FUNCTION "ASSE Z" : VOID
TITLE =GESTIONE SEGNALI DI STATO E COMANDO DELL'ASSE Z
VERSION : 0.1

BEGIN
NETWORK
TITLE =INS./DISIN.1
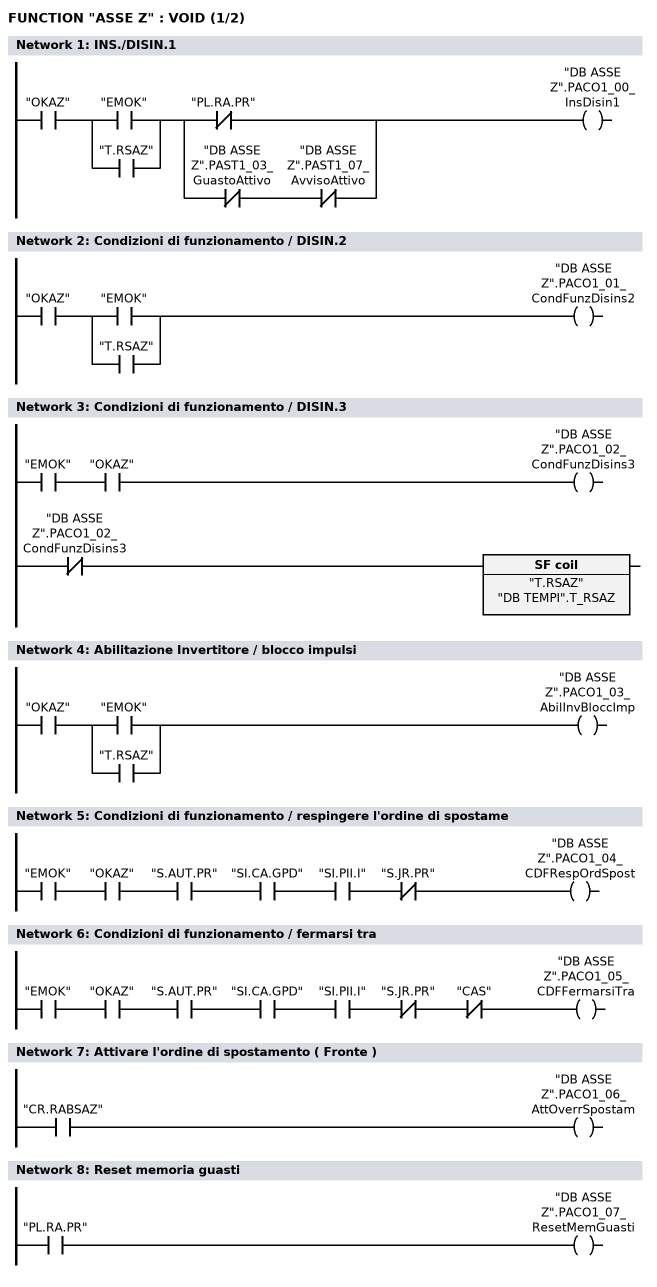
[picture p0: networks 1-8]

      U     "OKAZ";
      U(    ;
      O     "EMOK";
      O     "T.RSAZ";
      )     ;
      U(    ;
      UN    "PL.RA.PR";
      O     ;
      UN    "DB ASSE Z".PAST1_03_GuastoAttivo;
      UN    "DB ASSE Z".PAST1_07_AvvisoAttivo;
      )     ;
      =     "DB ASSE Z".PACO1_00_InsDisin1;

NETWORK
TITLE =Condizioni di funzionamento / DISIN.2

      U     "OKAZ";
      U(    ;
      O     "EMOK";
      O     "T.RSAZ";
      )     ;
      =     "DB ASSE Z".PACO1_01_CondFunzDisins2;

NETWORK
TITLE =Condizioni di funzionamento / DISIN.3

      U     "EMOK";
      U     "OKAZ";
      =     "DB ASSE Z".PACO1_02_CondFunzDisins3;
//---------------------------
      UN    "DB ASSE Z".PACO1_02_CondFunzDisins3;
      L     "DB TEMPI".T_RSAZ;
      SA    "T.RSAZ";

NETWORK
TITLE =Abilitazione Invertitore / blocco impulsi

      U     "OKAZ";
      U(    ;
      O     "EMOK";
      O     "T.RSAZ";
      )     ;
      =     "DB ASSE Z".PACO1_03_AbilInvBloccImp;

NETWORK
TITLE =Condizioni di funzionamento / respingere l'ordine di spostame

      U     "EMOK";
      U     "OKAZ";
      U     "S.AUT.PR";
      U     "SI.CA.GPD";
      U     "SI.PII.I";

      UN    "S.JR.PR";
      =     "DB ASSE Z".PACO1_04_CDFRespOrdSpost;

NETWORK
TITLE =Condizioni di funzionamento / fermarsi tra

      U     "EMOK";
      U     "OKAZ";
      U     "S.AUT.PR";
      U     "SI.CA.GPD";
      U     "SI.PII.I";
      UN    "S.JR.PR";

      UN    "CAS";
      =     "DB ASSE Z".PACO1_05_CDFFermarsiTra;

NETWORK
TITLE =Attivare l'ordine di spostamento ( Fronte )

      U     "CR.RABSAZ";
      =     "DB ASSE Z".PACO1_06_AttOverrSpostam;

NETWORK
TITLE =Reset memoria guasti

      U     "PL.RA.PR";
      =     "DB ASSE Z".PACO1_07_ResetMemGuasti;

NETWORK
TITLE =Marcia impulsi 1 INS
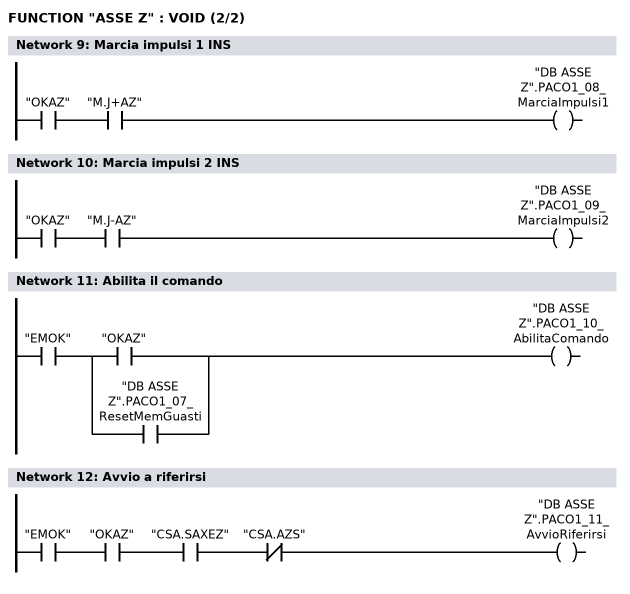
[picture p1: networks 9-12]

      U     "OKAZ";
      U     "M.J+AZ";
      =     "DB ASSE Z".PACO1_08_MarciaImpulsi1;

NETWORK
TITLE =Marcia impulsi 2 INS

      U     "OKAZ";
      U     "M.J-AZ";
      =     "DB ASSE Z".PACO1_09_MarciaImpulsi2;

NETWORK
TITLE =Abilita il comando

      U     "EMOK";
      U(    ;
      U     "OKAZ";
      O     ;
      U     "DB ASSE Z".PACO1_07_ResetMemGuasti;
      )     ;
      =     "DB ASSE Z".PACO1_10_AbilitaComando;

NETWORK
TITLE =Avvio a riferirsi

      U     "EMOK";
      U     "OKAZ";
      U     "CSA.SAXEZ";
      UN    "CSA.AZS";
      =     "DB ASSE Z".PACO1_11_AvvioRiferirsi;

NETWORK
TITLE =Cambio del blocco esterno

      CLR   ;
      =     "DB ASSE Z".PACO1_13_CambioBloccoExt;

NETWORK
TITLE =Caricamento del numero blocco di spostamento desiderato



NETWORK
TITLE =Funzionamento a seguire
//
      CLR   ;
      =     "DB ASSE Z".POSPACO_00_FunzASeguire;

NETWORK
TITLE =Imposta il punto di riferimento

      CLR   ;
      =     "DB ASSE Z".POSPACO_01_ImpostPuntRif;

NETWORK
TITLE =Camma di riferimento

      UN    "FC.ZAZ";
      =     "DB ASSE Z".POSPACO_02_CammaRiferime;

NETWORK
TITLE =Sensore della battuta fissa

      CLR   ;
      =     "DB ASSE Z".POSPACO_03_SensBattFissa;

NETWORK
TITLE =Attivare l'accoppiamento

      CLR   ;
      =     "DB ASSE Z".POSPACO_04_AttivAccoppia;

NETWORK
TITLE =Commutazione del blocco di parametri Bit 0

      CLR   ;
      =     "DB ASSE Z".PACO2_00_CommBlocParBit1;


NETWORK
TITLE =Commutazione del blocco di parametri Bit 1

      CLR   ;
      =     "DB ASSE Z".PACO2_01_CommBlocParBit2;

NETWORK
TITLE =Commutazione del blocco di parametri Bit 2

      CLR   ;
      =     "DB ASSE Z".PACO2_02_CommBlocParBit3;

NETWORK
TITLE =Primo filtro nel riferimento di velocita' disinserito
//
      CLR   ;
      =     "DB ASSE Z".PACO2_03_1FiltRifVelDisi;

NETWORK
TITLE =Tempo rampa zero

      CLR   ;
      =     "DB ASSE Z".PACO2_04_TempoRampaZero;

NETWORK
TITLE =Blocco dell'integratore nel regolatore di velocita'

      CLR   ;
      =     "DB ASSE Z".PACO2_06_BlocIntegrRegV;

NETWORK
TITLE =Scelta dell'asse in parcheggio

      CLR   ;
      =     "DB ASSE Z".PACO2_07_SceltaAsseInPar;

NETWORK
TITLE =Tacitare il guasto 608

      U     "OKAZ";
      U     "PL.RA.PR";
      =     "DB ASSE Z".PACO2_08_TacitGuasto608;

NETWORK
TITLE =Commutazione dati del motore 1 ingresso

      CLR   ;
      =     "DB ASSE Z".PACO2_09_CommDatiMot1Ing;

NETWORK
TITLE =Commutazione dati del motore 2 ingresso

      CLR   ;
      =     "DB ASSE Z".PACO2_10_CommDatiMot2Ing;

NETWORK
TITLE =Ha luogo la ommutazione del motore

      CLR   ;
      =     "DB ASSE Z".PACO2_11_CommutazMotore;

NETWORK
TITLE =OVERRIDE

      U     "M.MAN";
      UN    "P.JR.PR";
      SPBN  E001;
      L     "DB DATI".OVERRIDE_JOG;
      T     "DB ASSE Z".OVERRIDE;
      T     "DB DATI".OVERRIDE_ATTIVO;
E001: NOP   0;
      U     "M.MAN";
      U     "P.JR.PR";
      SPBN  E002;
      L     "DB DATI".OVERRIDE_JOG;
      L     2;
      *I    ;
      T     "DB ASSE Z".OVERRIDE;
      T     "DB DATI".OVERRIDE_ATTIVO;
E002: NOP   0;
      UN    "M.MAN";
      SPBN  E003;
      L     "DB DATI".OVERRIDE_AUT;
      T     "DB ASSE Z".OVERRIDE;
      T     "DB DATI".OVERRIDE_ATTIVO;
E003: NOP   0;

NETWORK
TITLE =Caricamento quote

      U     "ANSD";
      UN    "CQAZ.IC";
      S     "CQAZ.IC";
      S     "CQAZ.Q1";
//============================ QUOTA 1
      U     "CQAZ.Q1";
      SPBN  ET01;
      L     W#16#8051;
      T     "DB ASSE Z".PKE_Scrittura;
      L     W#16#1;
      T     "DB ASSE Z".IND_Scrittura;
      L     "DB QUOTE".Z_ATTESA;
      T     DB123.DBD    4;
//----------------------------
      U(    ;
      L     "DB ASSE Z".PKE_Lettura;
      L     W#16#5051;
      ==I   ;
      )     ;
      U(    ;
      L     "DB ASSE Z".IND_Lettura;
      L     W#16#1;
      ==I   ;
      )     ;
      R     "CQAZ.Q1";
      S     "CQAZ.Q2";
ET01: NOP   0;
//============================ QUOTA 2
      U     "CQAZ.Q2";
      SPBN  ET02;
      L     W#16#8051;
      T     "DB ASSE Z".PKE_Scrittura;
      L     W#16#2;
      T     "DB ASSE Z".IND_Scrittura;
      L     "DB QUOTE".Z_FUORI_INGOMBRO;
      T     DB123.DBD    4;
//----------------------------
      U(    ;
      L     "DB ASSE Z".PKE_Lettura;
      L     W#16#5051;
      ==I   ;
      )     ;
      U(    ;
      L     "DB ASSE Z".IND_Lettura;
      L     W#16#2;
      ==I   ;
      )     ;
      R     "CQAZ.Q2";
      S     "CQAZ.Q3";
ET02: NOP   0;
//============================ QUOTA 3
      U     "CQAZ.Q3";
      SPBN  ET03;
      L     W#16#8051;
      T     "DB ASSE Z".PKE_Scrittura;
      L     W#16#3;
      T     "DB ASSE Z".IND_Scrittura;
      L     "DB QUOTE".Z_DEPOSITO1;
      T     DB123.DBD    4;
//----------------------------
      U(    ;
      L     "DB ASSE Z".PKE_Lettura;
      L     W#16#5051;
      ==I   ;
      )     ;
      U(    ;
      L     "DB ASSE Z".IND_Lettura;
      L     W#16#3;
      ==I   ;
      )     ;
      R     "CQAZ.Q3";
      S     "CQAZ.Q4";
ET03: NOP   0;
//============================ QUOTA 4
      U     "CQAZ.Q4";
      SPBN  ET04;
      L     W#16#8051;
      T     "DB ASSE Z".PKE_Scrittura;
      L     W#16#4;
      T     "DB ASSE Z".IND_Scrittura;
      L     "DB QUOTE".Z_DEPOSITO2;
      T     DB123.DBD    4;
//----------------------------
      U(    ;
      L     "DB ASSE Z".PKE_Lettura;
      L     W#16#5051;
      ==I   ;
      )     ;
      U(    ;
      L     "DB ASSE Z".IND_Lettura;
      L     W#16#4;
      ==I   ;
      )     ;
      R     "CQAZ.Q4";
      S     "CQAZ.Q5";
ET04: NOP   0;
//============================ QUOTA 5
      U     "CQAZ.Q5";
      SPBN  ET05;
      L     W#16#8051;
      T     "DB ASSE Z".PKE_Scrittura;
      L     W#16#5;
      T     "DB ASSE Z".IND_Scrittura;
      L     "DB QUOTE".Z_DEPOSITO3;
      T     DB123.DBD    4;
//----------------------------
      U(    ;
      L     "DB ASSE Z".PKE_Lettura;
      L     W#16#5051;
      ==I   ;
      )     ;
      U(    ;
      L     "DB ASSE Z".IND_Lettura;
      L     W#16#5;
      ==I   ;
      )     ;
      R     "CQAZ.Q5";
      S     "CQAZ.Q6";
ET05: NOP   0;
//============================ QUOTA 6
      U     "CQAZ.Q6";
      SPBN  ET06;
      L     W#16#8051;
      T     "DB ASSE Z".PKE_Scrittura;
      L     W#16#6;
      T     "DB ASSE Z".IND_Scrittura;
      L     "DB QUOTE".Z_DEPOSITO4;
      T     DB123.DBD    4;
//----------------------------
      U(    ;
      L     "DB ASSE Z".PKE_Lettura;
      L     W#16#5051;
      ==I   ;
      )     ;
      U(    ;
      L     "DB ASSE Z".IND_Lettura;
      L     W#16#6;
      ==I   ;
      )     ;
      R     "CQAZ.Q6";
      S     "CQAZ.Q7";
ET06: NOP   0;
//============================ QUOTA 7
      U     "CQAZ.Q7";
      SPBN  ET07;
      L     W#16#8051;
      T     "DB ASSE Z".PKE_Scrittura;
      L     W#16#7;
      T     "DB ASSE Z".IND_Scrittura;
      L     "DB QUOTE".Z_DEPOSITO5;
      T     DB123.DBD    4;
//----------------------------
      U(    ;
      L     "DB ASSE Z".PKE_Lettura;
      L     W#16#5051;
      ==I   ;
      )     ;
      U(    ;
      L     "DB ASSE Z".IND_Lettura;
      L     W#16#7;
      ==I   ;
      )     ;
      R     "CQAZ.Q7";
      S     "CQAZ.Q8";
ET07: NOP   0;
//============================ QUOTA 8
      U     "CQAZ.Q8";
      SPBN  ET08;
      L     W#16#8051;
      T     "DB ASSE Z".PKE_Scrittura;
      L     W#16#8;
      T     "DB ASSE Z".IND_Scrittura;
      L     "DB QUOTE".Z_DEPOSITO6;
      T     DB123.DBD    4;
//----------------------------
      U(    ;
      L     "DB ASSE Z".PKE_Lettura;
      L     W#16#5051;
      ==I   ;
      )     ;
      U(    ;
      L     "DB ASSE Z".IND_Lettura;
      L     W#16#8;
      ==I   ;
      )     ;
      R     "CQAZ.Q8";
      S     "CQAZ.Q9";
ET08: NOP   0;
//============================ QUOTA 9
      U     "CQAZ.Q9";
      SPBN  ET09;
      L     W#16#8051;
      T     "DB ASSE Z".PKE_Scrittura;
      L     W#16#9;
      T     "DB ASSE Z".IND_Scrittura;
      L     "DB QUOTE".Z_DEPOSITO7;
      T     DB123.DBD    4;
//----------------------------
      U(    ;
      L     "DB ASSE Z".PKE_Lettura;
      L     W#16#5051;
      ==I   ;
      )     ;
      U(    ;
      L     "DB ASSE Z".IND_Lettura;
      L     W#16#9;
      ==I   ;
      )     ;
      R     "CQAZ.Q9";
      S     "CQAZ.Q10";
ET09: NOP   0;
//============================ QUOTA 10
      U     "CQAZ.Q10";
      SPBN  ET10;
      L     W#16#8051;
      T     "DB ASSE Z".PKE_Scrittura;
      L     W#16#A;
      T     "DB ASSE Z".IND_Scrittura;
      L     "DB QUOTE".Z_DEPOSITO8;
      T     DB123.DBD    4;
//----------------------------
      U(    ;
      L     "DB ASSE Z".PKE_Lettura;
      L     W#16#5051;
      ==I   ;
      )     ;
      U(    ;
      L     "DB ASSE Z".IND_Lettura;
      L     W#16#A;
      ==I   ;
      )     ;
      R     "CQAZ.Q10";
      S     "CQAZ.V1";
ET10: NOP   0;
//============================ VELOCITA' 1
      U     "CQAZ.V1";
      SPBN  ET11;
      L     W#16#8052;
      T     "DB ASSE Z".PKE_Scrittura;
      L     W#16#1;
      T     "DB ASSE Z".IND_Scrittura;
      L     "DB QUOTE".VELOCITA_Z;
      T     DB123.DBD    4;
//----------------------------
      U(    ;
      L     "DB ASSE Z".PKE_Lettura;
      L     W#16#5052;
      ==I   ;
      )     ;
      U(    ;
      L     "DB ASSE Z".IND_Lettura;
      L     W#16#1;
      ==I   ;
      )     ;
      R     "CQAZ.V1";
      S     "CQAZ.V2";
ET11: NOP   0;
//============================ VELOCITA' 2
      U     "CQAZ.V2";
      SPBN  ET12;
      L     W#16#8052;
      T     "DB ASSE Z".PKE_Scrittura;
      L     W#16#2;
      T     "DB ASSE Z".IND_Scrittura;
      L     "DB QUOTE".VELOCITA_Z;
      T     DB123.DBD    4;
//----------------------------
      U(    ;
      L     "DB ASSE Z".PKE_Lettura;
      L     W#16#5052;
      ==I   ;
      )     ;
      U(    ;
      L     "DB ASSE Z".IND_Lettura;
      L     W#16#2;
      ==I   ;
      )     ;
      R     "CQAZ.V2";
      S     "CQAZ.V3";
ET12: NOP   0;
//============================ VELOCITA' 3
      U     "CQAZ.V3";
      SPBN  ET13;
      L     W#16#8052;
      T     "DB ASSE Z".PKE_Scrittura;
      L     W#16#3;
      T     "DB ASSE Z".IND_Scrittura;
      L     "DB QUOTE".VELOCITA_Z;
      T     DB123.DBD    4;
//----------------------------
      U(    ;
      L     "DB ASSE Z".PKE_Lettura;
      L     W#16#5052;
      ==I   ;
      )     ;
      U(    ;
      L     "DB ASSE Z".IND_Lettura;
      L     W#16#3;
      ==I   ;
      )     ;
      R     "CQAZ.V3";
      S     "CQAZ.V4";
ET13: NOP   0;
//============================ VELOCITA' 4
      U     "CQAZ.V4";
      SPBN  ET14;
      L     W#16#8052;
      T     "DB ASSE Z".PKE_Scrittura;
      L     W#16#4;
      T     "DB ASSE Z".IND_Scrittura;
      L     "DB QUOTE".VELOCITA_Z;
      T     DB123.DBD    4;
//----------------------------
      U(    ;
      L     "DB ASSE Z".PKE_Lettura;
      L     W#16#5052;
      ==I   ;
      )     ;
      U(    ;
      L     "DB ASSE Z".IND_Lettura;
      L     W#16#4;
      ==I   ;
      )     ;
      R     "CQAZ.V4";
      S     "CQAZ.V5";
ET14: NOP   0;
//============================ VELOCITA' 5
      U     "CQAZ.V5";
      SPBN  ET15;
      L     W#16#8052;
      T     "DB ASSE Z".PKE_Scrittura;
      L     W#16#5;
      T     "DB ASSE Z".IND_Scrittura;
      L     "DB QUOTE".VELOCITA_Z;
      T     DB123.DBD    4;
//----------------------------
      U(    ;
      L     "DB ASSE Z".PKE_Lettura;
      L     W#16#5052;
      ==I   ;
      )     ;
      U(    ;
      L     "DB ASSE Z".IND_Lettura;
      L     W#16#5;
      ==I   ;
      )     ;
      R     "CQAZ.V5";
      S     "CQAZ.V6";
ET15: NOP   0;
//============================ VELOCITA' 6
      U     "CQAZ.V6";
      SPBN  ET16;
      L     W#16#8052;
      T     "DB ASSE Z".PKE_Scrittura;
      L     W#16#6;
      T     "DB ASSE Z".IND_Scrittura;
      L     "DB QUOTE".VELOCITA_Z;
      T     DB123.DBD    4;
//----------------------------
      U(    ;
      L     "DB ASSE Z".PKE_Lettura;
      L     W#16#5052;
      ==I   ;
      )     ;
      U(    ;
      L     "DB ASSE Z".IND_Lettura;
      L     W#16#6;
      ==I   ;
      )     ;
      R     "CQAZ.V6";
      S     "CQAZ.V7";
ET16: NOP   0;
//============================ VELOCITA' 7
      U     "CQAZ.V7";
      SPBN  ET17;
      L     W#16#8052;
      T     "DB ASSE Z".PKE_Scrittura;
      L     W#16#7;
      T     "DB ASSE Z".IND_Scrittura;
      L     "DB QUOTE".VELOCITA_Z;
      T     DB123.DBD    4;
//----------------------------
      U(    ;
      L     "DB ASSE Z".PKE_Lettura;
      L     W#16#5052;
      ==I   ;
      )     ;
      U(    ;
      L     "DB ASSE Z".IND_Lettura;
      L     W#16#7;
      ==I   ;
      )     ;
      R     "CQAZ.V7";
      S     "CQAZ.V8";
ET17: NOP   0;
//============================ VELOCITA' 8
      U     "CQAZ.V8";
      SPBN  ET18;
      L     W#16#8052;
      T     "DB ASSE Z".PKE_Scrittura;
      L     W#16#8;
      T     "DB ASSE Z".IND_Scrittura;
      L     "DB QUOTE".VELOCITA_Z;
      T     DB123.DBD    4;
//----------------------------
      U(    ;
      L     "DB ASSE Z".PKE_Lettura;
      L     W#16#5052;
      ==I   ;
      )     ;
      U(    ;
      L     "DB ASSE Z".IND_Lettura;
      L     W#16#8;
      ==I   ;
      )     ;
      R     "CQAZ.V8";
      S     "CQAZ.V9";
ET18: NOP   0;
//============================ VELOCITA' 9
      U     "CQAZ.V9";
      SPBN  ET19;
      L     W#16#8052;
      T     "DB ASSE Z".PKE_Scrittura;
      L     W#16#9;
      T     "DB ASSE Z".IND_Scrittura;
      L     "DB QUOTE".VELOCITA_Z;
      T     DB123.DBD    4;
//----------------------------
      U(    ;
      L     "DB ASSE Z".PKE_Lettura;
      L     W#16#5052;
      ==I   ;
      )     ;
      U(    ;
      L     "DB ASSE Z".IND_Lettura;
      L     W#16#9;
      ==I   ;
      )     ;
      R     "CQAZ.V9";
      S     "CQAZ.V10";
ET19: NOP   0;
//============================ VELOCITA' 10
      U     "CQAZ.V10";
      SPBN  ET20;
      L     W#16#8052;
      T     "DB ASSE Z".PKE_Scrittura;
      L     W#16#A;
      T     "DB ASSE Z".IND_Scrittura;
      L     "DB QUOTE".VELOCITA_Z;
      T     DB123.DBD    4;
//----------------------------
      U(    ;
      L     "DB ASSE Z".PKE_Lettura;
      L     W#16#5052;
      ==I   ;
      )     ;
      U(    ;
      L     "DB ASSE Z".IND_Lettura;
      L     W#16#A;
      ==I   ;
      )     ;
      R     "CQAZ.V10";
      S     "CQAZ.CT";
ET20: NOP   0;
      U     "CQAZ.CT";
      UN    "ANSD";
      R     "CQAZ.CT";
      R     "CQAZ.IC";

NETWORK
TITLE =Riduzione percentuale del limite di coppia

      L     0;
      T     "DB ASSE Z".MOMRID;

END_FUNCTION

